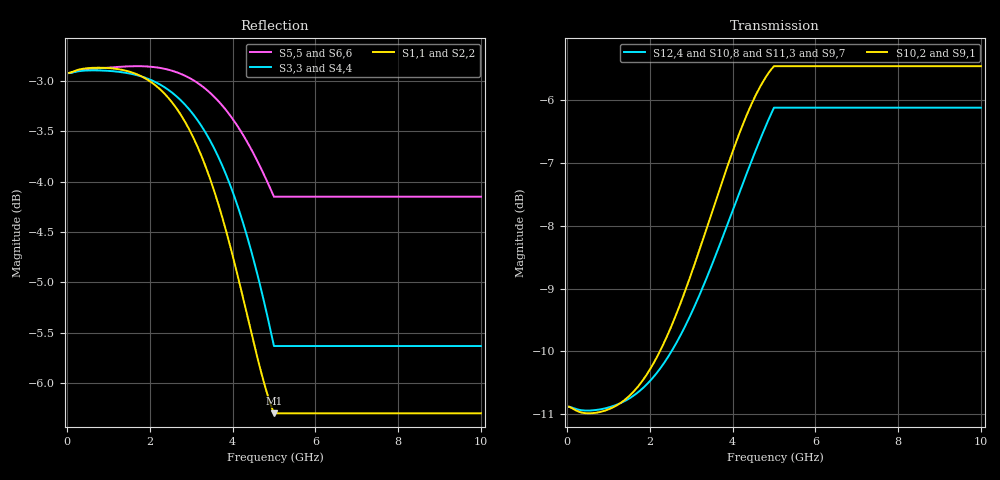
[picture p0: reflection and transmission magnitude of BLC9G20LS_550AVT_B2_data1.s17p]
! Created Tue Aug  4 23:43:13 2015
! 17 Port Network Data from SP1.SP block
! freq  magS1_1  angS1_1  magS1_2  angS1_2  magS1_3  angS1_3  magS1_4  angS1_4
!  magS1_5  angS1_5  magS1_6  angS1_6  magS1_7  angS1_7  magS1_8  angS1_8
!  magS1_9  angS1_9  magS1_10  angS1_10  magS1_11  angS1_11  magS1_12  angS1_12
!  magS1_13  angS1_13  magS1_14  angS1_14  magS1_15  angS1_15  magS1_16  angS1_16
!  magS1_17  angS1_17
!  magS2_1  angS2_1  magS2_2  angS2_2  magS2_3  angS2_3
!  magS2_4  angS2_4  magS2_5  angS2_5  magS2_6  angS2_6  magS2_7  angS2_7
!  magS2_8  angS2_8  magS2_9  angS2_9  magS2_10  angS2_10  magS2_11  angS2_11
!  magS2_12  angS2_12  magS2_13  angS2_13  magS2_14  angS2_14  magS2_15  angS2_15
!  magS2_16  angS2_16  magS2_17  angS2_17
!  magS3_1  angS3_1  magS3_2  angS3_2
!  magS3_3  angS3_3  magS3_4  angS3_4  magS3_5  angS3_5  magS3_6  angS3_6
!  magS3_7  angS3_7  magS3_8  angS3_8  magS3_9  angS3_9  magS3_10  angS3_10
!  magS3_11  angS3_11  magS3_12  angS3_12  magS3_13  angS3_13  magS3_14  angS3_14
!  magS3_15  angS3_15  magS3_16  angS3_16  magS3_17  angS3_17
!  magS4_1  angS4_1
!  magS4_2  angS4_2  magS4_3  angS4_3  magS4_4  angS4_4  magS4_5  angS4_5
!  magS4_6  angS4_6  magS4_7  angS4_7  magS4_8  angS4_8  magS4_9  angS4_9
!  magS4_10  angS4_10  magS4_11  angS4_11  magS4_12  angS4_12  magS4_13  angS4_13
!  magS4_14  angS4_14  magS4_15  angS4_15  magS4_16  angS4_16  magS4_17  angS4_17
!  magS5_1  angS5_1  magS5_2  angS5_2  magS5_3  angS5_3  magS5_4  angS5_4
!  magS5_5  angS5_5  magS5_6  angS5_6  magS5_7  angS5_7  magS5_8  angS5_8
!  magS5_9  angS5_9  magS5_10  angS5_10  magS5_11  angS5_11  magS5_12  angS5_12
!  magS5_13  angS5_13  magS5_14  angS5_14  magS5_15  angS5_15  magS5_16  angS5_16
!  magS5_17  angS5_17
!  magS6_1  angS6_1  magS6_2  angS6_2  magS6_3  angS6_3
!  magS6_4  angS6_4  magS6_5  angS6_5  magS6_6  angS6_6  magS6_7  angS6_7
!  magS6_8  angS6_8  magS6_9  angS6_9  magS6_10  angS6_10  magS6_11  angS6_11
!  magS6_12  angS6_12  magS6_13  angS6_13  magS6_14  angS6_14  magS6_15  angS6_15
!  magS6_16  angS6_16  magS6_17  angS6_17
!  magS7_1  angS7_1  magS7_2  angS7_2
!  magS7_3  angS7_3  magS7_4  angS7_4  magS7_5  angS7_5  magS7_6  angS7_6
!  magS7_7  angS7_7  magS7_8  angS7_8  magS7_9  angS7_9  magS7_10  angS7_10
!  magS7_11  angS7_11  magS7_12  angS7_12  magS7_13  angS7_13  magS7_14  angS7_14
!  magS7_15  angS7_15  magS7_16  angS7_16  magS7_17  angS7_17
!  magS8_1  angS8_1
!  magS8_2  angS8_2  magS8_3  angS8_3  magS8_4  angS8_4  magS8_5  angS8_5
!  magS8_6  angS8_6  magS8_7  angS8_7  magS8_8  angS8_8  magS8_9  angS8_9
!  magS8_10  angS8_10  magS8_11  angS8_11  magS8_12  angS8_12  magS8_13  angS8_13
!  magS8_14  angS8_14  magS8_15  angS8_15  magS8_16  angS8_16  magS8_17  angS8_17
!  magS9_1  angS9_1  magS9_2  angS9_2  magS9_3  angS9_3  magS9_4  angS9_4
!  magS9_5  angS9_5  magS9_6  angS9_6  magS9_7  angS9_7  magS9_8  angS9_8
!  magS9_9  angS9_9  magS9_10  angS9_10  magS9_11  angS9_11  magS9_12  angS9_12
!  magS9_13  angS9_13  magS9_14  angS9_14  magS9_15  angS9_15  magS9_16  angS9_16
!  magS9_17  angS9_17
!  magS10_1  angS10_1  magS10_2  angS10_2  magS10_3  angS10_3
!  magS10_4  angS10_4  magS10_5  angS10_5  magS10_6  angS10_6  magS10_7  angS10_7
!  magS10_8  angS10_8  magS10_9  angS10_9  magS10_10  angS10_10  magS10_11  angS10_11
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# ghz S ma R 50
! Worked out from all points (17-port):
!   200 points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, 50 MHz to 10 GHz, reference 50 ohm
!   strongest paths, dB at 50 MHz, 2.55 GHz, 5.05 GHz, 7.55 GHz, 10 GHz:
!     S10,2: -10.9, -9.6, -5.5, -5.5, -5.5
!     S9,1: -10.9, -9.6, -5.5, -5.5, -5.5
!     S12,4: -10.9, -10.0, -6.1, -6.1, -6.1
!     S10,8: -10.9, -10.1, -6.2, -6.2, -6.2
!     S11,3: -10.9, -10.0, -6.2, -6.2, -6.2
!     S9,7: -10.9, -10.2, -6.2, -6.2, -6.2
!   lowest |S11| = -6.3 dB at 5 GHz (marker M1), VSWR 2.88, Z = 17.4 + j1.84 ohm
!   |S11| at or under -10 dB: nowhere
